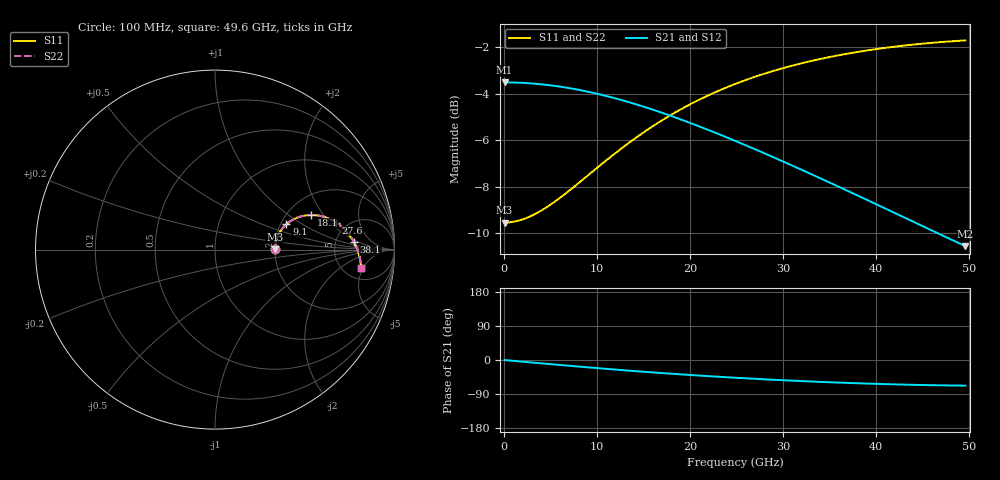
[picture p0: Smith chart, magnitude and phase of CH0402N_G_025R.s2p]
# GHz S RI R 25
! S-Parameters data
! Freq  reS11  imS11  reS21  imS21  reS12  imS12  reS22  imS22
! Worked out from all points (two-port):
!   100 points, 100 MHz to 49.6 GHz, reference 25 ohm
!   highest |S21| = -3.52 dB at 100 MHz (marker M1); lowest = -10.6 dB at 49.6 GHz (marker M2)
!   |S21| within 3 dB of the highest: start of sweep to 27.75 GHz
!   lowest |S11| = -9.5 dB at 100 MHz (marker M3), VSWR 2.00, Z = 50 + j0.199 ohm
!   |S11| at or under -10 dB: nowhere
!   |S22| runs from -9.5 to -1.7 dB; largest |S21 - S12| = 0
!   S11 on the Smith chart (normalised r, x): 100 MHz: 2.00, +0.01; 9.1 GHz: 2.15, +0.74; 18.1 GHz: 2.68, +1.53; 27.6 GHz: 4.07, +2.35; 38.1 GHz: 7.57, +1.58; 49.6 GHz: 7.31, -4.51
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0.1  0.3333 0.00177  0.6667 -0.00256  0.6667 -0.00256  0.3333 0.00177
1.6  0.3355 0.0282  0.6644 -0.0408  0.6644 -0.0408  0.3355 0.0282
3.6  0.3442 0.0624  0.6554 -0.0907  0.6554 -0.0907  0.3442 0.0624
6.1  0.3636 0.1016  0.6352 -0.1495  0.6352 -0.1495  0.3636 0.1016
8.6  0.3912 0.1352  0.6065 -0.2026  0.6065 -0.2026  0.3912 0.1352
9.1  0.3976 0.141  0.5999 -0.2124  0.5999 -0.2124  0.3976 0.141
11.1  0.4251 0.1615  0.5711 -0.2485  0.5711 -0.2485  0.4251 0.1615
13.1  0.4553 0.1768  0.5394 -0.2794  0.5394 -0.2794  0.4553 0.1768
14.6  0.4791 0.1849  0.5143 -0.2992  0.5143 -0.2992  0.4791 0.1849
16.6  0.5116 0.1912  0.48 -0.321  0.48 -0.321  0.5116 0.1912
18.1  0.5359 0.1927  0.454 -0.3342  0.454 -0.3342  0.5359 0.1927
19.6  0.5601 0.1917  0.4282 -0.3447  0.4282 -0.3447  0.5601 0.1917
21.6  0.5913 0.1866  0.3944 -0.3551  0.3944 -0.3551  0.5913 0.1866
25.1  0.6424 0.1689  0.3384 -0.3641  0.3384 -0.3641  0.6424 0.1689
27.6  0.6752 0.1506  0.3016 -0.3648  0.3016 -0.3648  0.6752 0.1506
30.6  0.71 0.1237  0.2616 -0.3606  0.2616 -0.3606  0.71 0.1237
33.1  0.735 0.0983  0.2318 -0.3539  0.2318 -0.3539  0.735 0.0983
35.6  0.7564 0.0707  0.2052 -0.3449  0.2052 -0.3449  0.7564 0.0707
38.1  0.7743 0.0415  0.1819 -0.3342  0.1819 -0.3342  0.7743 0.0415
41.6  0.7936 -0.00102  0.1544 -0.3172  0.1544 -0.3172  0.7936 -0.00102
45.6  0.8078 -0.0509  0.1301 -0.2961  0.1301 -0.2961  0.8078 -0.0509
49.6  0.814 -0.1009  0.1129 -0.2744  0.1129 -0.2744  0.814 -0.1009
